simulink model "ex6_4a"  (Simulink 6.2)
settings: Solver=VariableStepDiscrete  SolverMode=SingleTasking  StartTime=0.0  StopTime=1.0  RelTol=1e-3  AbsTol=1e-6

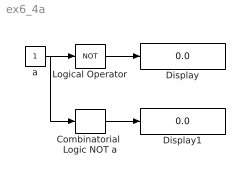
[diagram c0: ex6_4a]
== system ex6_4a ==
  Combinatorial  Logic NOT a : CombinatorialLogic  TruthTable=[1;0]
  Display : Display
  Display1 : Display
  Logical Operator : Logic  Operator=NOT  Inputs=1
  a : Constant
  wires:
  a/1 -> Combinatorial  Logic NOT a/1, Logical Operator/1
  Combinatorial  Logic NOT a/1 -> Display1/1
  Logical Operator/1 -> Display/1
